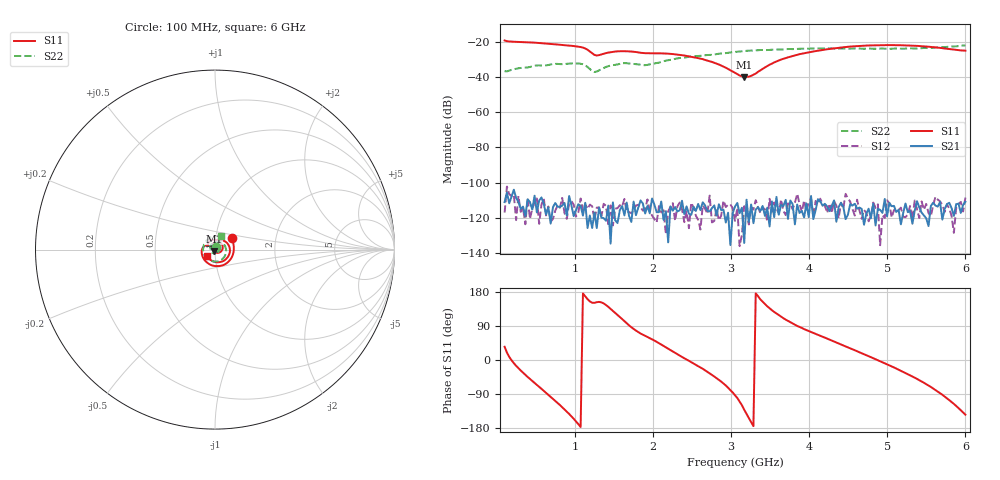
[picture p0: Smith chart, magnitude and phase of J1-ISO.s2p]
!Agilent Technologies,E8364B,MY43040379,A.07.50.67
!Agilent E8364B: A.07.50.67
!Date: Tuesday, March 24, 2026 11:35:12
!Correction: S11(Full 2 Port(1,2))
!S21(Full 2 Port(1,2))
!S12(Full 2 Port(1,2))
!S22(Full 2 Port(1,2))
!S2P File: Measurements: S11, S21, S12, S22:
# Hz S  dB  R 50
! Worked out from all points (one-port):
!   201 points, 100 MHz to 6 GHz, reference 50 ohm
!   lowest |S11| = -39.7 dB at 3.168 GHz (marker M1), VSWR 1.02, Z = 49.3 - j0.764 ohm
!   |S11| at or under -10 dB: start of sweep to end of sweep
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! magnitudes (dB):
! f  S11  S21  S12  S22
! 100 MHz  -18.9  -111.2  -117.1  -36.5
! 513 MHz  -20.3  -117.1  -109.1  -33.2
! 749 MHz  -21.1  -111.7  -116.1  -32.3
! 1.103 GHz  -23.0  -118.9  -116.0  -32.5
! 1.25 GHz  -27.2  -117.1  -121.3  -36.9
! 1.427 GHz  -25.8  -113.1  -123.8  -33.6
! 1.605 GHz  -25.0  -113.4  -113.7  -32.0
! 1.899 GHz  -26.2  -117.7  -115.2  -33.0
! 2.076 GHz  -26.2  -116.9  -113.4  -31.6
! 2.312 GHz  -27.0  -116.5  -113.6  -29.1
! 2.637 GHz  -29.6  -111.3  -113.1  -27.5
! 2.844 GHz  -32.6  -112.4  -121.4  -26.5
! 3.05 GHz  -37.3  -113.7  -121.9  -25.5
! 3.168 GHz  -39.7  -134.5  -113.5  -24.9
! 3.256 GHz  -39.1  -112.5  -113.9  -24.7
! 3.493 GHz  -32.7  -125.1  -109.3  -24.3
! 3.64 GHz  -29.8  -112.8  -109.7  -24.1
! 4.053 GHz  -25.2  -120.9  -119.1  -23.5
! 4.525 GHz  -22.4  -112.3  -110.9  -23.6
! 5.027 GHz  -21.6  -111.6  -111.9  -23.7
! 5.469 GHz  -22.3  -118.8  -115.5  -23.2
! 6 GHz  -24.7  -111.0  -108.6  -21.7
